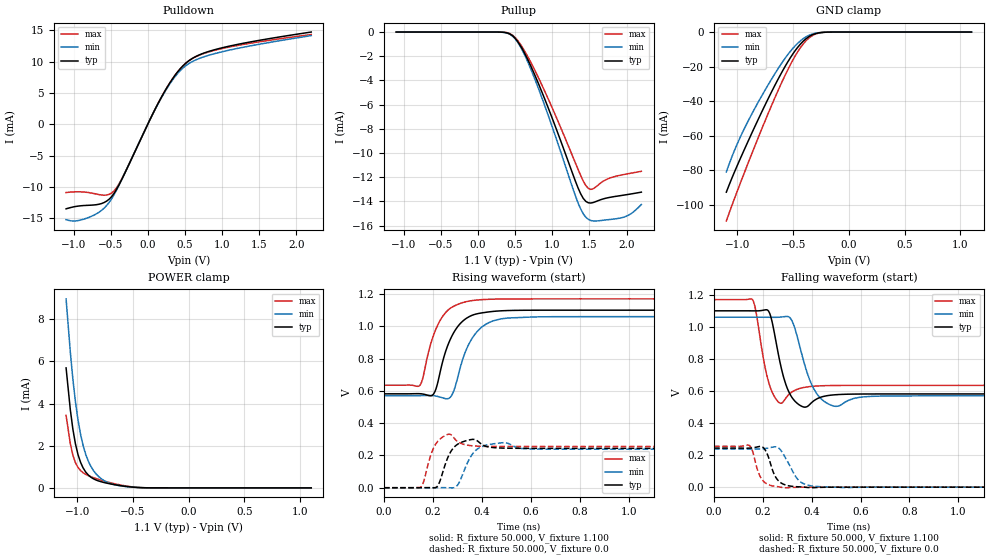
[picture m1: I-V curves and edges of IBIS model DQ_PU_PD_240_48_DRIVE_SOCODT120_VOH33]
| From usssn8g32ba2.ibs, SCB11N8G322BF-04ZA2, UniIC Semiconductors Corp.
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|   Model DQ_PU_PD_240_48_DRIVE_SOCODT120_VOH33
[Model] DQ_PU_PD_240_48_DRIVE_SOCODT120_VOH33
Model_type I/O
Polarity   Inverting
Vinl =  98.000mV
Vinh =  0.268V
Vmeas =  0.183V
Rref =  50.000
Vref =  0.183V
C_comp   1.020pF   1.010pF   1.030pF
[Model Spec]
Vinh   0.268V   0.262V   0.280V
Vinl   98.000mV   92.000mV   0.110V
Vmeas   0.183V   0.177V   0.195V
Vref   0.183V   0.177V   0.195V
Rref   50.000   NA   NA
[Temperature Range]   25.000   0.105k   -40.000
[Voltage Range]   1.100V   1.060V   1.170V
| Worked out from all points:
|   slope of the pulldown table from 0 to 0.165 V, typ, clamps not added: 42.3 ohm
|   GND clamp passes 1 mA (typ) near -0.30 V on its own axis
|   POWER clamp passes 1 mA (typ) near -0.95 V on its own axis
|   rising waveform, R_fixture 50.000, V_fixture 1.100: 20-80 % time 75.3ps typ, 78.9ps min, 72.6ps max; typ from 0.582 V to 1.1 V
|   rising waveform, R_fixture 50.000, V_fixture 0.0: 20-80 % time 32.8ps typ, 41.8ps min, 27.1ps max; typ from 0 V to 0.244 V
|   falling waveform, R_fixture 50.000, V_fixture 1.100: 20-80 % time 42.4ps typ, 55.5ps min, 34.4ps max; typ from 1.1 V to 0.582 V
|   falling waveform, R_fixture 50.000, V_fixture 0.0: 20-80 % time 37.7ps typ, 54.5ps min, 33.4ps max; typ from 0.244 V to 0 V
[Pulldown]
|Voltage   I(typ)   I(min)   I(max)
-1.1V     -13.51mA   -15.24mA   -10.91mA
-930mV    -13.06mA   -15.37mA   -10.79mA
-726mV    -12.89mA   -14.52mA   -11.06mA
-556mV    -12.29mA   -13.01mA   -11.31mA
-454mV    -11.04mA   -11.25mA   -10.65mA
-318mV    -8.03mA    -8.027mA   -7.964mA
158mV     3.751mA    3.687mA    3.768mA
328mV     7.153mA    6.973mA    7.158mA
498mV     9.598mA    9.214mA    9.581mA
668mV     10.93mA    10.37mA    10.89mA
940mV     12.01mA    11.39mA    11.91mA
2.2V      14.71mA    14.14mA    14.31mA
[Pullup]
|Voltage   I(typ)   I(min)   I(max)
-1.1V     1nA        10.92nA    0A
432mV     -168.8uA   -190.8uA   -131.8uA
568mV     -1.092mA   -1.17mA    -975.3uA
704mV     -2.706mA   -2.942mA   -2.412mA
942mV     -6.202mA   -6.816mA   -5.469mA
1.316V    -12.39mA   -13.6mA    -10.88mA
1.452V    -13.99mA   -15.3mA    -12.68mA
1.554V    -14.09mA   -15.62mA   -12.95mA
1.724V    -13.73mA   -15.53mA   -12.2mA
1.928V    -13.51mA   -15.36mA   -11.82mA
2.064V    -13.38mA   -15mA      -11.66mA
2.2V      -13.23mA   -14.25mA   -11.51mA
[GND_clamp]
|Voltage   I(typ)   I(min)   I(max)
-1.1V     -92.78mA   -81.05mA   -109.5mA
-1.031V   -81.73mA   -69.22mA   -97.17mA
-939mV    -68.18mA   -56.02mA   -81.64mA
-824mV    -52mA      -41.83mA   -62.83mA
-686mV    -33.62mA   -26.41mA   -41.32mA
-571mV    -19.76mA   -15.06mA   -24.85mA
-479mV    -10.5mA    -7.76mA    -13.5mA
-410mV    -5.313mA   -3.84mA    -6.916mA
-341mV    -2.007mA   -1.45mA    -2.59mA
-272mV    -506.9uA   -403.5uA   -609.8uA
-180mV    -45.65uA   -51.35uA   -43.55uA
1.1V      0A         0A         0A
[POWER_clamp]
|Voltage   I(typ)   I(min)   I(max)
-1.1V     5.691mA    8.967mA    3.44mA
-1.062V   3.709mA    6.444mA    2.092mA
-1.039V   2.781mA    5.152mA    1.546mA
-1.016V   2.086mA    4.085mA    1.193mA
-970mV    1.21mA     2.539mA    818.5uA
-947mV    943.7uA    2.005mA    716.7uA
-901mV    610.1uA    1.27mA     581.3uA
-855mV    430.7uA    824.1uA    484.6uA
-786mV    289.9uA    439.4uA    366uA
-671mV    155.9uA    155.9uA    203.6uA
-441mV    13.2uA     12.79uA    15.03uA
1.1V      0A         0A         0A
[Ramp]
| variable   typ   min   max
dV/dt_r   0.146/32.887p   0.143/41.912p   0.153/27.186p
dV/dt_f   0.311/42.584p   0.294/55.707p   0.321/34.400p
R_load = 50.000
[Rising Waveform]
R_fixture= 50.000
V_fixture= 1.100
V_fixture_min= 1.060
V_fixture_max= 1.170
|time   V(typ)   V(min)   V(max)
0s        581.6mV    569.9mV    635mV
146ps     582.5mV    570.5mV    633.7mV
208ps     595.4mV    568.9mV    967.8mV
265ps     899.6mV    553.7mV    1.105V
285ps     961.7mV    600.6mV    1.125V
313ps     1.02V      753.7mV    1.143V
369ps     1.073V     946.3mV    1.161V
448ps     1.093V     1.035V     1.168V
593ps     1.1V       1.057V     1.17V
3ns       1.1V       1.06V      1.17V
[Rising Waveform]
R_fixture= 50.000
V_fixture= 0.0
V_fixture_min= 0.0
V_fixture_max= 0.0
|time   V(typ)   V(min)   V(max)
0s        2.898uV    10.6uV     685nV
151ps     144.4uV    23.29uV    4.611mV
194ps     279.5uV    102.7uV    215mV
217ps     7.212mV    336.3uV    283mV
265ps     202.1mV    -128.7uV   331.6mV
300ps     268.7mV    16.12mV    286.4mV
381ps     290.4mV    239.8mV    257.7mV
485ps     245.4mV    278.8mV    255.2mV
607ps     244mV      239.7mV    255mV
3ns       243.9mV    238.7mV    255mV
[Falling Waveform]
R_fixture= 50.000
V_fixture= 1.100
V_fixture_min= 1.060
V_fixture_max= 1.170
|time   V(typ)   V(min)   V(max)
0s        1.1V       1.06V      1.17V
158ps     1.1V       1.06V      1.167V
224ps     1.096V     1.06V      651.9mV
273ps     757.8mV    1.061V     523.3mV
314ps     571.5mV    1.05V      588.3mV
355ps     507.5mV    853.6mV    617.5mV
419ps     549.4mV    586.3mV    630.9mV
499ps     576.7mV    504mV      634.3mV
693ps     581.5mV    568.6mV    635mV
3ns       581.6mV    569.9mV    635mV
[Falling Waveform]
R_fixture= 50.000
V_fixture= 0.0
V_fixture_min= 0.0
V_fixture_max= 0.0
|time   V(typ)   V(min)   V(max)
0s        243.9mV    238.7mV    255mV
144ps     243.6mV    238.4mV    260.1mV
155ps     244.9mV    238.2mV    236.1mV
198ps     250.8mV    239mV      44.61mV
217ps     209.3mV    242.6mV    19.88mV
253ps     60.52mV    251.6mV    4.664mV
292ps     13.92mV    183.2mV    -4.089mV
349ps     2.138mV    39.09mV    -522.4uV
436ps     -1.143mV   2.872mV    -16.76uV
3ns       2.829uV    10.68uV    500.5nV
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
